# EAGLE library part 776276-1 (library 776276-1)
8POS,PIN DIA 1.3,HDR ASSY,180DEG,SLDR,AMPSEAL, Automotive Headers, Wire-to-Board / Wire-to-Device, 8 Position, 4mm [.157in] Centerline, Sealable, Vertical, 3 Row, Black Source: Datasheet
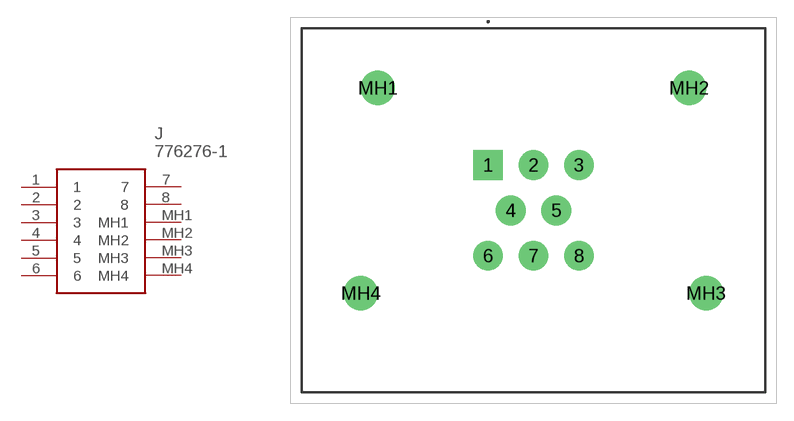
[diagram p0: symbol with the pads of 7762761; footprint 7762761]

Designator prefix J

## 776276-1 (Description: 8POS,PIN DIA 1.3,HDR ASSY,180DEG,SLDR,AMPSEAL, Automotive Headers, Wire-to-Board / Wire-to-Device, 8 Position, 4mm [.157in] Centerline, Sealable, Vertical, 3 Row, Black; Height: 34.5mm; Manufacturer_Name: TE Connectivity; Manufacturer_Part_Number: 776276-1; Mouser_Part_Number: 571-776276-1; Mouser_Price-Stock: https://www.mouser.co.uk/ProductDetail/TE-Connectivity/776276-1?qs=tLAa1RwIH6dOXUCPhsBe4Q%3D%3D)  [7762761]
1  1
2  2
3  3
4  4
5  5
6  6
7  7
8  8
MH1  MH1
MH2  MH2
MH3  MH3
MH4  MH4

## Footprint 7762761 (pad centres in mm)
776276-1-2
drill 1.75 pad 2.625 square: 1 0,0
drill 1.75 pad 2.625: 2 4,0; 3 8,0; 4 2,-4; 5 6,-4; 6 0,-8; 7 4,-8; 8 8,-8
drill 2 pad 3: MH1 -9.7,6.8; MH2 17.7,6.8; MH3 19.2,-11.3; MH4 -11.2,-11.3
